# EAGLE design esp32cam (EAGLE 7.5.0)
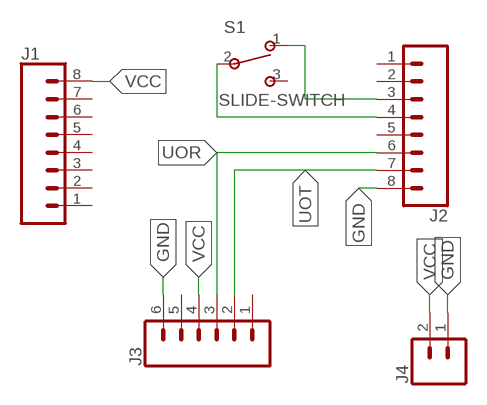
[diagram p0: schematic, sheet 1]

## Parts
J1  CONN_08"  [1X08]
J2  CONN_08"  [1X08]
J3  CONN_06LOCK  [1X06_LOCK]
J4  CONN_02  [1X02]
S1  SLIDE-SWITCH  [AYZ0102AGRLC]

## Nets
GND: J2.8 J3.6 J4.1
N$1: J2.3 S1.1
N$6: J2.4 S1.2
UOR: J2.6 J3.3
UOT: J2.7 J3.2
VCC: J1.8 J3.4 J4.2
Unconnected: J1.1 J1.2 J1.3 J1.4 J1.5 J1.6 J1.7 J2.1 J2.2 J2.5 J3.1 J3.5 S1.3

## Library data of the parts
J1 J2 = SparkFun-Connectors:CONN_08: Multi connection point. Often used as Generic Header-pin footprint for 0.1 inch spaced/style header connections On any of the 0.1 inch spaced packages, you can populate with these: Break Away Headers - Straight (PRT-00116) Break Away Male Headers - Right Angle (PRT-00553) Female Headers (PRT-00115)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; PROD_ID: CONN-08438
J3 = SparkFun-Connectors:CONN_06: Multi connection point. Often used as Generic Header-pin footprint for 0.1 inch spaced/style header connections On any of the 0.1 inch spaced packages, you can populate with these: Break Away Headers - Straight (PRT-00116) Break Away Male Headers - Right Angle (PRT-00553) Female Headers (PRT-00115)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
J4 = SparkFun-Connectors:CONN_02: Multi connection point. Often used as Generic Header-pin footprint for 0.1 inch spaced/style header connections
S1 = fab:SLIDE-SWITCH: SMD slide-switch AYZ0102AGRLC as found in the fablab inventory. Includes the mounting holes. Made by Zaerc.

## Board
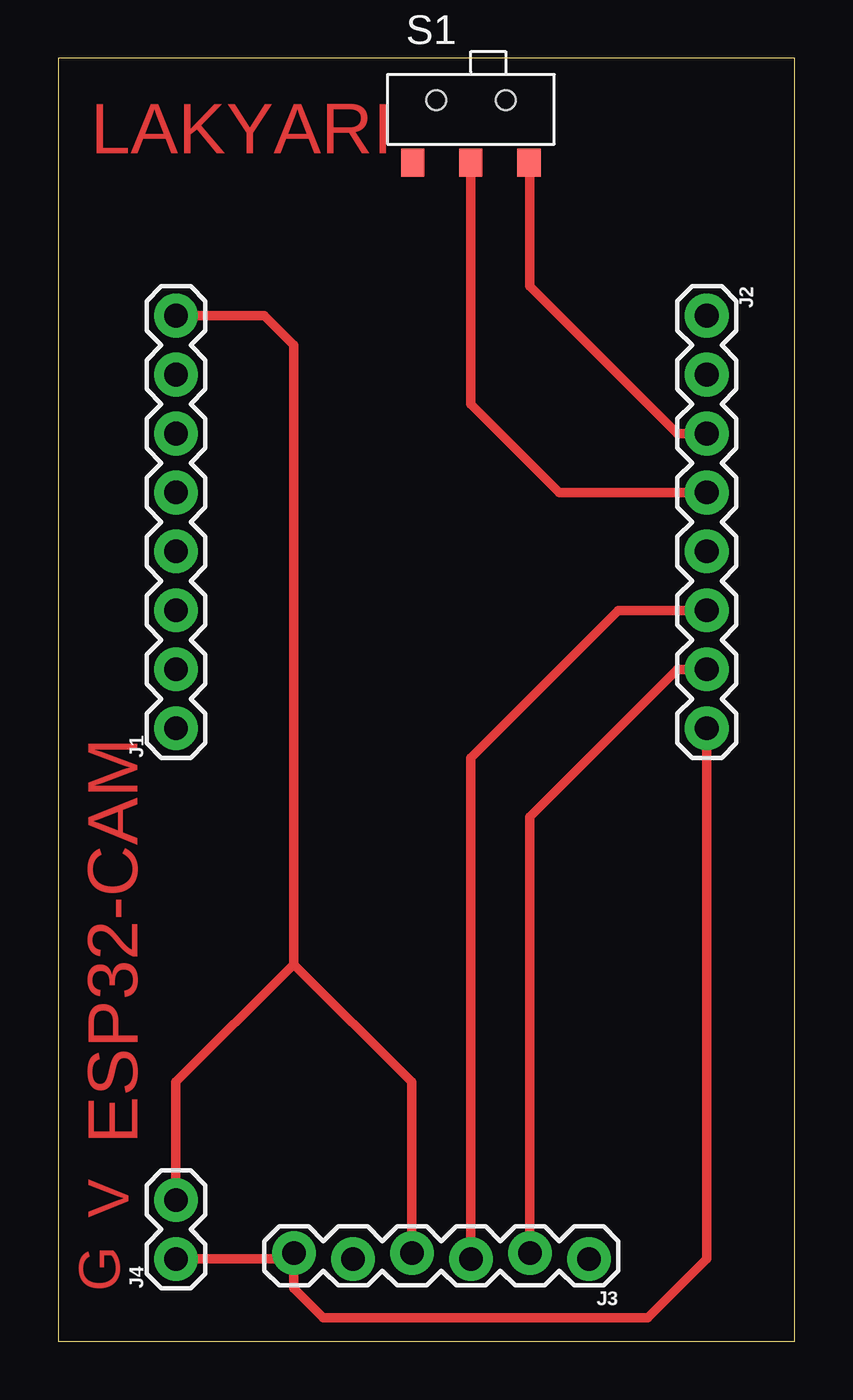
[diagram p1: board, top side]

Size 31.73 x 55.3 mm. Coordinates in mm from the lower left corner, seen from the top.
Outline: 0,0 31.73,0 31.73,55.3 0,55.3 0,0
Copper layers (1*16): Top 0.035mm / dielectric 1.5mm / Bottom 0.035mm
Design rules "default": minimum track width 10mil, minimum drill 24mil, track to track 8mil, track to pad 8mil, pad to pad 8mil, via to via 8mil, smd to smd 8mil, copper to edge 40mil, drill to drill 8mil, minimum pad ring 10mil, minimum via ring 8mil, stop-mask expansion 4mil, vias tented up to drill 0mil, thermal gap 10mil

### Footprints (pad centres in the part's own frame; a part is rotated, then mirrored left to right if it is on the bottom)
1X08 = drill 1.016 pad 1.88: 1 0,0; 2 2.54,0; 3 5.08,0; 4 7.62,0; 5 10.16,0; 6 12.7,0; 7 15.24,0; 8 17.78,0
1X06_LOCK = drill 1.016 pad 1.88: 1 0,0; 2 2.54,-0.254; 3 5.08,0; 4 7.62,-0.254; 5 10.16,0; 6 12.7,-0.254
1X02 = drill 1.016 pad 1.88: 1 0,0; 2 2.54,0
AYZ0102AGRLC = smd 1 x 1.2: 1 2.5,-2.3; 2 0,-2.3; 3 -2.5,-2.3 | hole 0.85: -1.5,0.4; 1.5,0.4

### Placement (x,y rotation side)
J1  5.08,26.42 90 top
J2  27.94,44.2 270 top
J3  22.86,3.56 180 top
J4  5.08,3.56 90 top
S1  17.78,53.09 0 top

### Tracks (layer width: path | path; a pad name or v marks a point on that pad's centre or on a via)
GND
  Top 0.406: J2.8 27.94,3.56 25.4,1.02 11.43,1.02 10.16,2.29 J3.6 9.91,3.56 J4.1
N$1
  Top 0.406: J2.3 26.67,39.12 20.32,45.47 20.32,50.75 S1.1
N$6
  Top 0.406: S1.2 17.78,40.39 21.59,36.58 J2.4
UOR
  Top 0.406: J2.6 24.13,31.5 17.78,25.15 J3.3
UOT
  Top 0.406: J2.7 26.67,28.96 20.32,22.61 J3.2
VCC
  Top 0.406: J1.8 8.89,44.2 10.16,42.93 10.16,16.26 | 10.16,16.26 15.24,11.18 J3.4 | J4.2 5.08,11.18 10.16,16.26

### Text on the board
Top: LAKYARI | ESP32-CAM | V | G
